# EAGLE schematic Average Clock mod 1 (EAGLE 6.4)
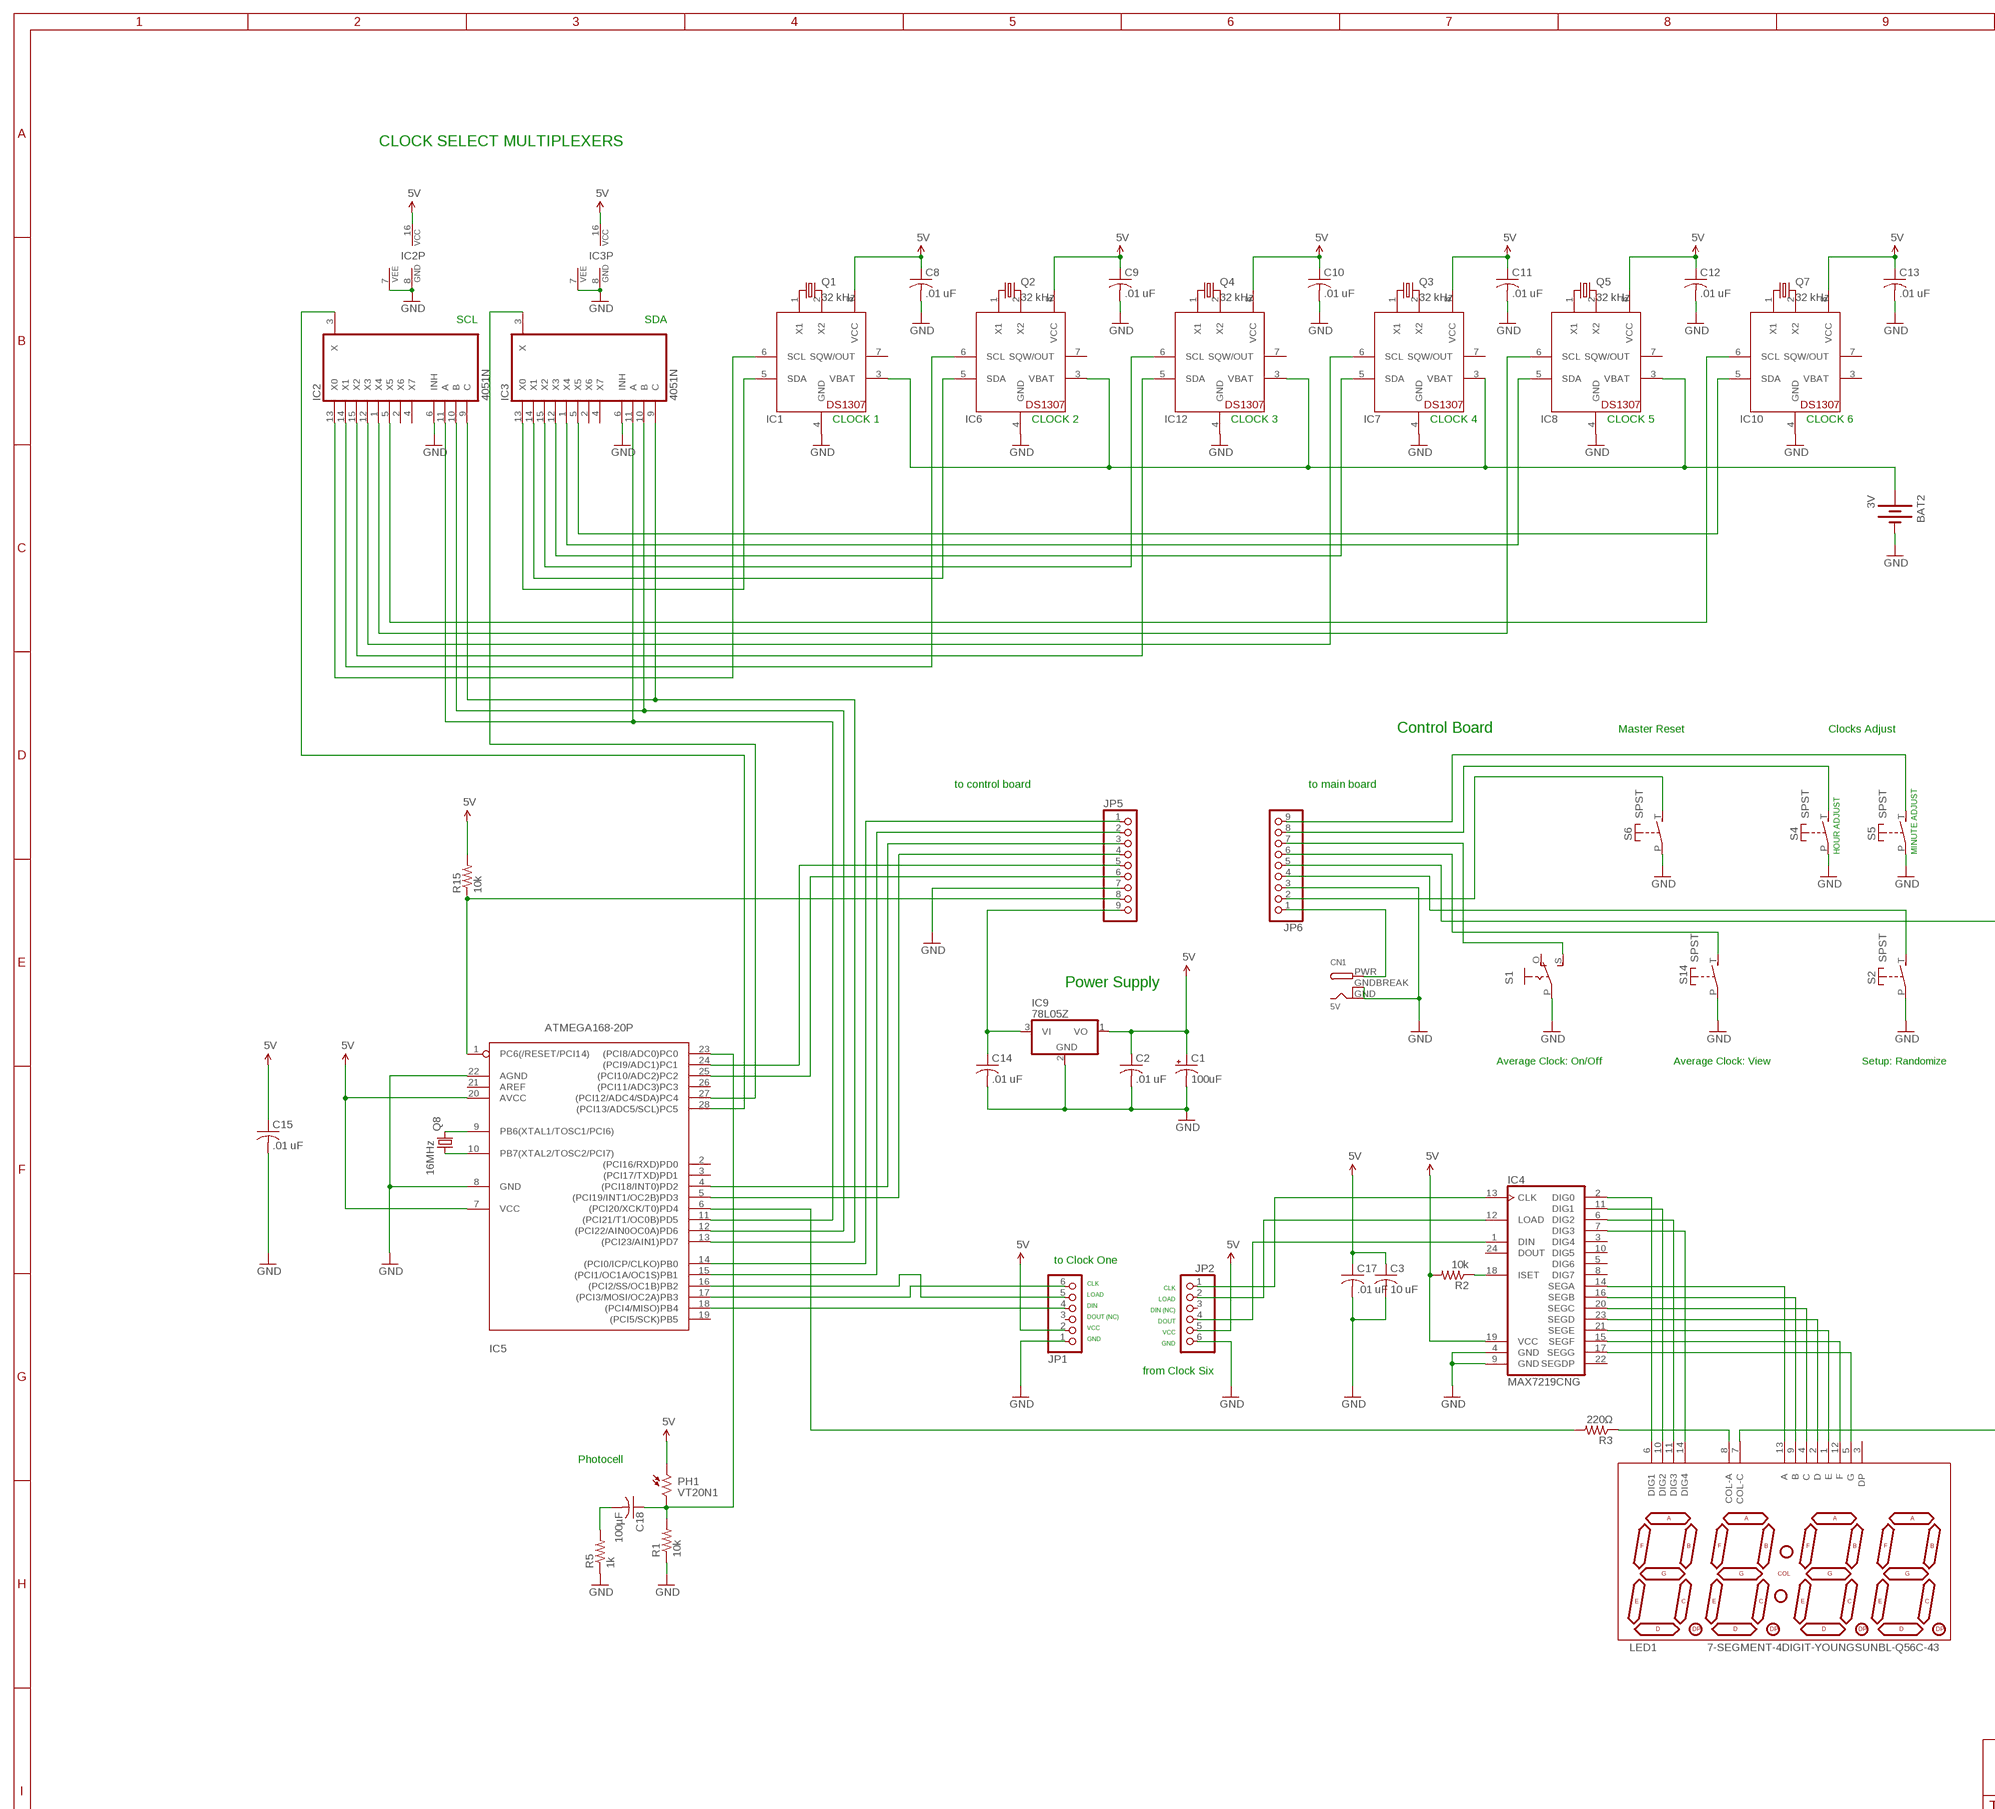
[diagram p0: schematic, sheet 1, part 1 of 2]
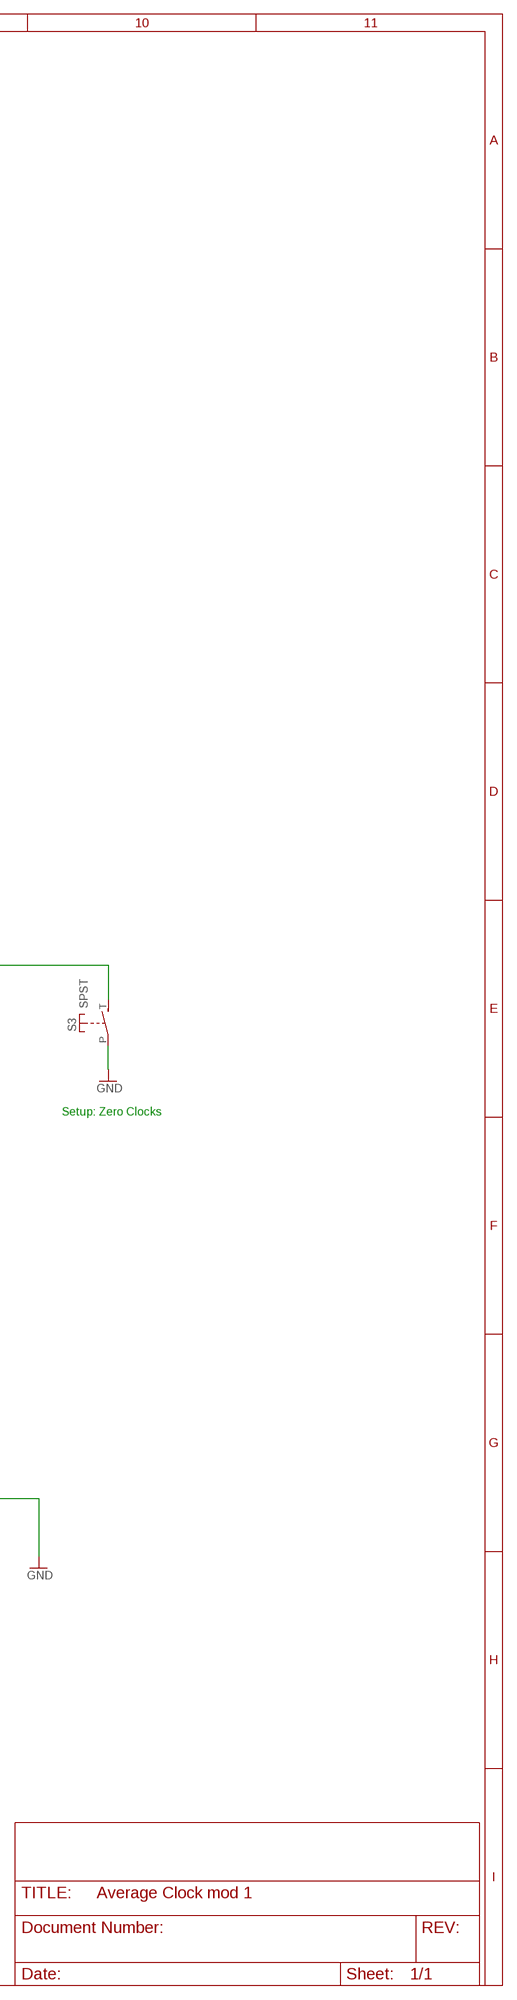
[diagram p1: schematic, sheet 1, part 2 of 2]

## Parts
BAT2  3V  BATTERY20PTH  [BATTCOM_20MM_PTH]
C1  100uF  CPOL-USE2,5-6E  [E2,5-6E]
C2  .01 uF  C-US025-025X050  [C025-025X050]
C3  10 uF  C-US025-025X050  [C025-025X050]
C8  .01 uF  C-US025-025X050  [C025-025X050]
C9  .01 uF  C-US025-025X050  [C025-025X050]
C10  .01 uF  C-US025-025X050  [C025-025X050]
C11  .01 uF  C-US025-025X050  [C025-025X050]
C12  .01 uF  C-US025-025X050  [C025-025X050]
C13  .01 uF  C-US025-025X050  [C025-025X050]
C14  .01 uF  C-US025-025X050  [C025-025X050]
C15  .01 uF  C-US025-025X050  [C025-025X050]
C17  .01 uF  C-US025-025X050  [C025-025X050]
C18  100µF  C-US025-024X044  [C025-024X044]
CN1  5V  DCBARRELPTH  [DCJACK_2MM_PTH]
IC1  DS1307  [DIL08]
IC2  4051N  [DIL16]
IC3  4051N  [DIL16]
IC4  MAX7219CNG  [DIL24-3]
IC5  ATMEGA168-20P  [DIL28-3]
IC6  DS1307  [DIL08]
IC7  DS1307  [DIL08]
IC8  DS1307  [DIL08]
IC9  78L05Z  [TO92]
IC10  DS1307  [DIL08]
IC12  DS1307  [DIL08]
JP1  PINHD-1X6  [1X06]
JP2  PINHD-1X6  [1X06]
JP5  PINHD-1X9  [1X09-BIG]
JP6  PINHD-1X9  [1X09-BIG]
LED1  7-SEGMENT-4DIGIT-YOUNGSUNBL-Q56C-43  [7-SEGMENT-4DIGIT-YOUNGSUN]
PH1  VT20N1  [TO46-VT200]
Q1  32 kHz  CRYSTALTC26H  [TC26H]
Q2  32 kHz  CRYSTALTC26H  [TC26H]
Q3  32 kHz  CRYSTALTC26H  [TC26H]
Q4  32 kHz  CRYSTALTC26H  [TC26H]
Q5  32 kHz  CRYSTALTC26H  [TC26H]
Q7  32 kHz  CRYSTALTC26H  [TC26H]
Q8  16MHz  CRYSTALHC49S  [HC49/S]
R1  10k  R-US_0204/5  [0204/5]
R2  10k  R-US_0204/5  [0204/5]
R3  220Ω  R-US_0204/5  [0204/5]
R5  1k  R-US_0204/5  [0204/5]
R15  10k  R-US_0204/5  [0204/5]
S1  EG1218S  [EG1218]
S2  SPST  [JUDCOSPST]
S3  SPST  [JUDCOSPST]
S4  SPST  [JUDCOSPST]
S5  SPST  [JUDCOSPST]
S6  SPST  [JUDCOSPST]
S14  SPST  [JUDCOSPST]

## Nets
5V: C1.+ C2.1 C3.1 C8.1 C9.1 C10.1 C11.1 C12.1 C13.1 C15.1 C17.1 IC1.8(VCC) IC2.16(VCC) IC3.16(VCC) IC4.19(VCC) IC5.7(VCC) IC5.20(AVCC) IC6.8(VCC) IC7.8(VCC) IC8.8(VCC) IC9.1(VO) IC10.8(VCC) IC12.8(VCC) JP1.2 JP2.5 PH1.1 R2.2 R15.2
GND: BAT2.2(-) C1.- C2.2 C3.2 C8.2 C9.2 C10.2 C11.2 C12.2 C13.2 C14.2 C15.2 C17.2 CN1.GND CN1.GNDBREAK IC1.4(GND) IC2.6(INH) IC2.7(VEE) IC2.8(GND) IC3.6(INH) IC3.7(VEE) IC3.8(GND) IC4.4(GND) IC4.9(GND) IC5.8(GND) IC5.22(AGND) IC6.4(GND) IC7.4(GND) IC8.4(GND) IC9.2(GND) IC10.4(GND) IC12.4(GND) JP1.1 JP2.6 JP5.7 JP6.3 LED1.7(COL-C) R1.1 R5.1 S1.P S2.P S3.P S4.P S5.P S6.P S14.P
N$1: IC8.2(X2) Q5.2
N$2: IC3.3(X) IC5.27((PCI12/ADC4/SDA)PC4)
N$3: LED1.8(COL-A) R3.1
N$5: IC1.2(X2) Q1.2
N$6: IC1.1(X1) Q1.1
N$7: IC6.2(X2) Q2.2
N$8: IC6.1(X1) Q2.1
N$9: IC7.2(X2) Q3.2
N$10: IC7.1(X1) Q3.1
N$11: BAT2.1(+) IC1.3(VBAT) IC6.3(VBAT) IC7.3(VBAT) IC8.3(VBAT) IC12.3(VBAT)
N$12: IC1.5(SDA) IC3.13(X0)
N$13: IC3.14(X1) IC6.5(SDA)
N$14: IC1.6(SCL) IC2.13(X0)
N$15: IC2.14(X1) IC6.6(SCL)
N$16: IC2.15(X2) IC12.5(SDA)
N$17: IC3.15(X2) IC12.6(SCL)
N$18: IC4.2(DIG0) LED1.6(DIG1)
N$19: IC4.11(DIG1) LED1.10(DIG2)
N$20: IC4.6(DIG2) LED1.11(DIG3)
N$21: IC5.9(PB6(XTAL1/TOSC1/PCI6)) Q8.2
N$22: IC4.7(DIG3) LED1.14(DIG4)
N$23: IC4.14(SEGA) LED1.13(A)
N$24: IC4.16(SEGB) LED1.9(B)
N$25: IC4.20(SEGC) LED1.4(C)
N$26: JP6.8 S4.T(S)
N$27: IC8.1(X1) Q5.1
N$28: IC2.3(X) IC5.28((PCI13/ADC5/SCL)PC5)
N$29: IC12.2(X2) Q4.2
N$30: IC12.1(X1) Q4.1
N$31: IC2.12(X3) IC7.6(SCL)
N$32: IC3.12(X3) IC7.5(SDA)
N$33: JP6.7 S1.S
N$34: C18.1 IC5.23((PCI8/ADC0)PC0) PH1.2 R1.2
N$35: IC5.10(PB7(XTAL2/TOSC2/PCI7)) Q8.1
N$36: IC4.18(ISET) R2.1
N$37: IC2.1(X4) IC8.6(SCL)
N$38: IC3.5(X5) IC10.5(SDA)
N$39: IC3.1(X4) IC8.5(SDA)
N$40: IC2.5(X5) IC10.6(SCL)
N$41: IC4.23(SEGD) LED1.2(D)
N$42: IC4.21(SEGE) LED1.1(E)
N$43: IC4.15(SEGF) LED1.12(F)
N$44: IC4.17(SEGG) LED1.5(G)
N$45: IC10.2(X2) Q7.2
N$46: IC10.1(X1) Q7.1
N$47: C14.1 IC9.3(VI) JP5.9
N$48: IC5.6((PCI20/XCK/T0)PD4) R3.2
N$49: JP6.6 S14.T(S)
N$50: C18.2 R5.2
N$51: IC5.18((PCI4/MISO)PB4) JP1.4
N$52: IC5.16((PCI2/SS/OC1B)PB2) JP1.5
N$53: JP6.9 S5.T(S)
N$54: IC4.12(LOAD) JP2.2
N$55: IC4.13(CLK) JP2.1
N$56: IC5.17((PCI3/MOSI/OC2A)PB3) JP1.6
N$57: IC2.9(C) IC3.9(C) IC5.13((PCI23/AIN1)PD7)
N$58: IC2.10(B) IC3.10(B) IC5.12((PCI22/AIN0OC0A)PD6)
N$59: IC2.11(A) IC3.11(A) IC5.11((PCI21/T1/OC0B)PD5)
N$60: IC5.25((PCI10/ADC2)PC2) JP5.6
N$61: IC5.24((PCI9/ADC1)PC1) JP5.5
N$62: IC5.1(PC6(/RESET/PCI14)) JP5.8 R15.1
N$63: IC5.14((PCI0/ICP/CLKO)PB0) JP5.1
N$64: CN1.PWR JP6.1
N$65: IC4.1(DIN) JP2.4
N$66: IC5.15((PCI1/OC1A/OC1S)PB1) JP5.2
N$67: IC5.4((PCI18/INT0)PD2) JP5.3
N$68: IC5.5((PCI19/INT1/OC2B)PD3) JP5.4
N$69: JP6.5 S3.T(S)
N$70: JP6.2 S6.T(S)
N$71: JP6.4 S2.T(S)
Unconnected: IC1.7(SQW/OUT) IC2.2(X6) IC2.4(X7) IC3.2(X6) IC3.4(X7) IC4.3(DIG4) IC4.5(DIG6) IC4.8(DIG7) IC4.10(DIG5) IC4.22(SEGDP) IC4.24(DOUT) IC5.2((PCI16/RXD)PD0) IC5.3((PCI17/TXD)PD1) IC5.19((PCI5/SCK)PB5) IC5.21(AREF) IC5.26((PCI11/ADC3)PC3) IC6.7(SQW/OUT) IC7.7(SQW/OUT) IC8.7(SQW/OUT) IC10.7(SQW/OUT) IC12.7(SQW/OUT) JP1.3 JP2.3 LED1.3(DP) S1.O

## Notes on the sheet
- CLOCK SELECT MULTIPLEXERS
- SCL | SDA
- CLOCK 1 | CLOCK 2 | CLOCK 3 | CLOCK 4 | CLOCK 5 | CLOCK 6
- Control Board | Master Reset | Clocks Adjust
- to control board | to main board
- HOUR ADJUST | MINUTE ADJUST
- Power Supply
- Average Clock: On/Off | Average Clock: View | Setup: Randomize | Setup: Zero Clocks
- to Clock One
- CLK | CLK
- LOAD | LOAD
- DIN | DIN (NC)
- DOUT (NC) | DOUT
- VCC | VCC
- GND | GND
- from Clock Six
- Photocell

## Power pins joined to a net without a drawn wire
VBAT: IC10.3(VBAT)

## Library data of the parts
BAT2 = SparkFun:BATTERY: Battery Holders
C1 = adafruit:CPOL-US: POLARIZED CAPACITOR, American symbol
C2 C3 C8-C15 C17 = rcl:C-US: CAPACITOR, American symbol
C18 = adafruit:C-US: CAPACITOR, American symbol
CN1 = adafruit:DCBARREL: 2.0mm DC Barrel Jack DCJACK_2MM_PTH - Through Hole Jack (4UConnector: 05537)
IC1 IC6-IC8 IC10 IC12 = adafruit:DS1307: DS1307 Real time clock (RTC) with battery backup ability. Talk to it via i2c
IC2 IC3 = 40xx:4051: 8-channel ANALOG MULTIPLEXER
IC4 = maxim:MAX7219CNG: LED DISPLAY DRIVER; MF: MAXIM; MPN: MAX7219CNG; OC_FARNELL: 1523914; OC_NEWARK: 34C4018
IC5 = adafruit:ATMEGA168*P: MICROCONTROLLER 16 kBytes FLASH 1 kBytes SRAM 512 Bytes EEPROM USART 8-channel 10 bit ADC
IC9 = adafruit:78*: Positive VOLTAGE REGULATOR Added bigger pads to the TO-92 package
JP1 JP2 = adafruit:PINHD-1X6: PIN HEADER
JP5 JP6 = adafruit:PINHD-1X9: Pin header 1x10 0.1" spacing With round pins
LED1 = BL-Q56x43old:7-SEGMENT-4DIGIT-YOUNGSUN: This is a part for the 4-Digit 7-segment LEDs from Young Sun. Different from the Digikey LEDs, all 16 pins are used. The LONGPADS Variant is used for a test jig, but you may like it because there is more pad to solder to. If you are concerned about routing space, the standard works just fine though.
PH1 = photo-elements:VT2*: Photoconductive Cell VT200 Series
Q1-Q5 Q7 = crystal:CRYSTAL: CRYSTAL; OC_FARNELL: unknown; OC_NEWARK: unknown
Q8 = crystal:CRYSTAL: CRYSTAL; OC_FARNELL: 1667008; OC_NEWARK: unknown
R1-R3 R5 R15 = rcl:R-US_: RESISTOR, American symbol
S1 = adafruit:EG1218: SLIDING SWITCH 0.1" spacing through hole, vertical SPDT slide switch http://www.ladyada.net/library/pcb/eaglelibrary.html
S2-S6 S14 = adafruit:SPST: Judco 50-0015-00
